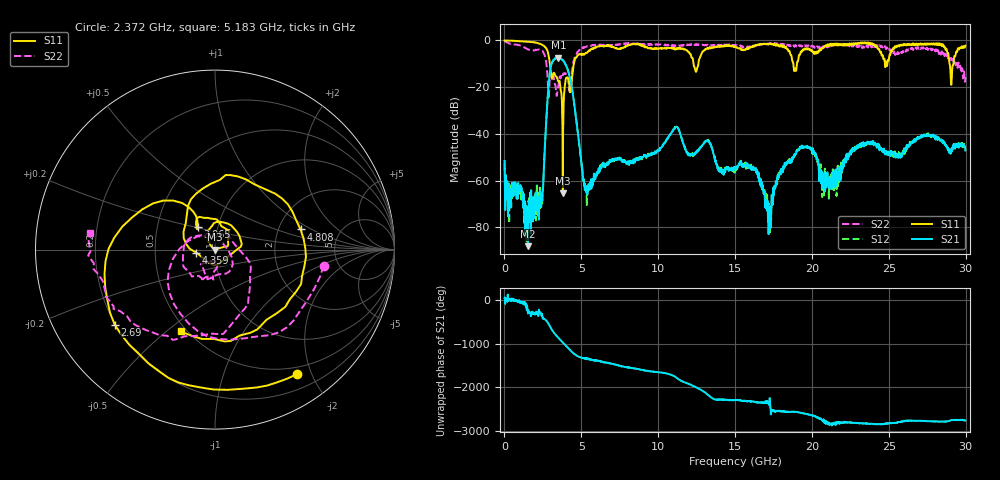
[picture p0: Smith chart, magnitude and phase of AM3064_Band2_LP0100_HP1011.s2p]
# Hz S DB R 50.0
!freq dBS11 angS11 dBS21 angS21 dBS12 angS12 dBS22 angS22
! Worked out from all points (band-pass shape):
!   1600 points, 10 MHz to 29.98 GHz, reference 50 ohm
!   highest |S21| = -7.40 dB at 3.515 GHz (marker M1); lowest = -88.0 dB at 1.528 GHz (marker M2)
!   |S21| within 3 dB of the highest: 3.045 GHz to 3.976 GHz (931.3 MHz wide, 26.5 % of centre)
!   lowest |S11| = -65.3 dB at 3.796 GHz (marker M3), VSWR 1.00, Z = 50 + j0.0415 ohm
!   |S11| at or under -10 dB: 2.954 GHz to 4.514 GHz (1.56 GHz wide, 41.8 % of centre); 12.3 GHz to 12.61 GHz (310.2 MHz wide, 2.49 % of centre); 28.95 GHz to 29.2 GHz (257.6 MHz wide, 0.886 % of centre)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
!   |S22| runs from -25.1 to -0.2 dB; largest |S21 - S12| = 0.0099
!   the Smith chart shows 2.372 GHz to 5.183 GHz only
!   S11 on the Smith chart (normalised r, x): 2.372 GHz: 0.40, -1.78; 2.69 GHz: 0.20, -0.32; 3.065 GHz: 0.80, +0.20; 4.359 GHz: 0.81, -0.03; 4.808 GHz: 2.65, +0.78; 5.183 GHz: 0.47, -0.56
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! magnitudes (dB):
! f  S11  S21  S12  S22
! 10 MHz  -0.1  -51.6  -52.7  -0.2
! 1.528 GHz  -0.6  -88.0  -71.1  -3.8
! 2.372 GHz  -1.6  -68.4  -65.6  -4.3
! 2.69 GHz  -3.1  -37.8  -37.7  -8.4
! 3.065 GHz  -16.1  -10.0  -9.9  -17.1
! 3.515 GHz  -17.6  -7.4  -7.5  -19.2
! 3.796 GHz  -65.3  -8.5  -8.4  -14.9
! 4.359 GHz  -19.6  -19.3  -19.2  -14.6
! 4.808 GHz  -6.2  -41.3  -41.2  -4.6
! 5.015 GHz  -6.3  -52.3  -53.6  -3.8
! 5.183 GHz  -6.1  -61.2  -61.6  -3.1
! 10 GHz  -3.5  -47.1  -47.0  -1.8
! 11.2 GHz  -3.6  -37.0  -37.0  -2.3
! 15 GHz  -2.6  -55.4  -54.8  -1.9
! 16.37 GHz  -2.1  -55.6  -56.0  -2.2
! 17.22 GHz  -1.4  -74.0  -75.2  -1.5
! 18.14 GHz  -3.0  -55.1  -54.9  -1.8
! 19.99 GHz  -4.3  -46.9  -46.6  -2.3
! 20.98 GHz  -2.2  -61.6  -60.6  -3.0
! 23.2 GHz  -1.2  -44.7  -45.1  -2.5
! 25 GHz  -8.3  -48.3  -48.6  -3.3
! 29.98 GHz  -2.3  -47.1  -46.1  -15.7
